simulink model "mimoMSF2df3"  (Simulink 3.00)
settings: Solver=ode45  StartTime=0.0  StopTime=50.0  RelTol=1e-3
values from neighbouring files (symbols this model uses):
  Disturb = Setpoint    [mimo_MSF1DF_sim.m]    (also in mimo_MSF2DF_sim.m)
  K = 1/kpd    [imc2pseucon.m]    (also in imc2pseudo.m)
  Satlb = temp1    [cback.m]    (also in imcmenu.m = str2num(satlbs))
  Satub = temp1    [cback.m]    (also in imcmenu.m = str2num(satubs))
  Setpoint = zeros(1,n)    [mimo_MSF1DF_sim.m]    (also in mimo_MSF2DF_sim.m)
undefined symbols (not defined in the file or in its folder): Ds, input_delay, Kdelay, Ksp, T
libraries: MIMO_lib x14, simulink3 x12

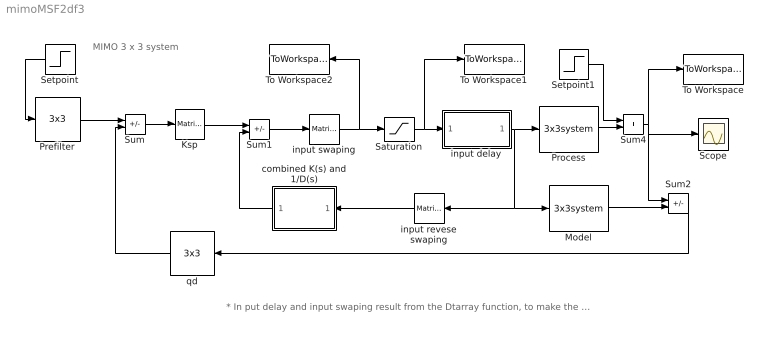
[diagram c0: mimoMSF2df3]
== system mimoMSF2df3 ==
  note: * In put delay and input swaping result from the Dtarray function, to make the system be able to be decoupled.
  note: MIMO 3 x 3 system
  Ksp : simulink3/Math/Matrix Gain  K=Ksp
  Model : MIMO_lib/3x3system  num=Mnum  den=Mden  dead=Mdead
  Prefilter : MIMO_lib/3x3  num=prefilnum  den=prefilden
  Process : MIMO_lib/3x3system  num=Pnum  den=Pden  dead=Pdead
  Saturation : Saturate  UpperLimit=Satub  LowerLimit=Satlb
  Scope : Scope
  Setpoint : Step  Orientation=left  Time=0  Before=0  After=[Setpoint]  SampleTime=0
  Setpoint1 : Step  Time=0  Before=0  After=[Disturb]  SampleTime=0
  Sum : Sum  Inputs=+-  SaturateOnIntegerOverflow=on
  Sum1 : Sum  Inputs=+-  SaturateOnIntegerOverflow=on
  Sum2 : Sum  Inputs=+-  SaturateOnIntegerOverflow=on
  Sum4 : Sum  Inputs=++  SaturateOnIntegerOverflow=on
  To Workspace : ToWorkspace  VariableName=yout  SampleTime=0  SaveFormat=Matrix
  To Workspace1 : ToWorkspace  VariableName=sat_effort  SampleTime=0  SaveFormat=Matrix
  To Workspace2 : ToWorkspace  VariableName=unsat_effort  SampleTime=0  SaveFormat=Matrix
  combined K(s) and 1/D(s) : Subsystem  Orientation=left  mask(ksds){Ksp=Ksp, Ds=Ds, Kdelay=Kdelay, K=K}
      mask prompts: Ds "D(s)"; Kdelay "Bdelay"; K "B*(s)"
  input delay : Subsystem  mask(input delay){input_delay=input_delay}
      mask prompts: input_delay "Input Delay (vector)"
  input revese swaping : simulink3/Math/Matrix Gain  Orientation=left  K=T
  input swaping : simulink3/Math/Matrix Gain  K=inv(T)
  qd : MIMO_lib/3x3  Orientation=left  num=qdnum  den=qdden
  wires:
  Ksp/1 -> Sum1/1
  combined K(s) and 1/D(s)/1(Out1) -> Sum1/2
  Sum/1 -> Ksp/1
  input revese swaping/1 -> combined K(s) and 1/D(s)/1(In1)
  Model/1 -> Sum2/2
  Process/1 -> Sum4/2
  Setpoint1/1 -> Sum4/1
  Sum4/1 -> Sum2/1, To Workspace/1, Scope/1
  input swaping/1 -> Saturation/1, To Workspace2/1
  Sum1/1 -> input swaping/1
  input delay/1(Out1) -> Process/1, Model/1, input revese swaping/1
  Saturation/1 -> input delay/1(In1), To Workspace1/1
  Prefilter/1 -> Sum/1
  Setpoint/1 -> Prefilter/1
  Sum2/1 -> qd/1
  qd/1 -> Sum/2

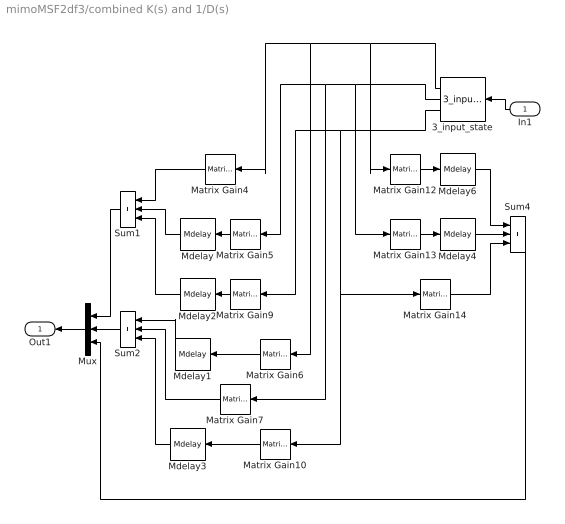
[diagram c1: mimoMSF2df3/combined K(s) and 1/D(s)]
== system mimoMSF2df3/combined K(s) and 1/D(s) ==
  In1 : Inport  Orientation=left  Port=1  PortWidth=-1  SampleTime=-1  DataType=auto
  3_input_state : MIMO_lib/3_input_state  Orientation=left  Ds=Ds
  Matrix Gain10 : simulink3/Math/Matrix Gain  Orientation=left  K="[zeros(1,length(Ds{3})-length(K{2,3}))  K{2,3}]"
  Matrix Gain12 : simulink3/Math/Matrix Gain  K="[zeros(1,length(Ds{1})-length(K{3,1}))  K{3,1}]"
  Matrix Gain13 : simulink3/Math/Matrix Gain  K="[zeros(1,length(Ds{2})-length(K{3,2}))  K{3,2}]"
  Matrix Gain14 : simulink3/Math/Matrix Gain  K="[zeros(1,length(Ds{3})-length(K{3,3}))  K{3,3}]"
  Matrix Gain4 : simulink3/Math/Matrix Gain  Orientation=left  K="[zeros(1,length(Ds{1})-length(K{1,1}))  K{1,1}]"
  Matrix Gain5 : simulink3/Math/Matrix Gain  Orientation=left  K=[zeros(1,length(Ds{2})-length(K{1,2})) K{1,2}]
  Matrix Gain6 : simulink3/Math/Matrix Gain  Orientation=left  K="[zeros(1,length(Ds{1})-length(K{2,1}))  K{2,1}]"
  Matrix Gain7 : simulink3/Math/Matrix Gain  Orientation=left  K="[zeros(1,length(Ds{2})-length(K{2,2}))  K{2,2}]"
  Matrix Gain9 : simulink3/Math/Matrix Gain  Orientation=left  K="[zeros(1,length(Ds{3})-length(K{1,3}))  K{1,3}]"
  Mdelay : MIMO_lib/Mdelay  Orientation=left  Mdelay=Kdelay(1,2)
  Mdelay1 : MIMO_lib/Mdelay  Orientation=left  Mdelay=Kdelay(2,1)
  Mdelay2 : MIMO_lib/Mdelay  Orientation=left  Mdelay=Kdelay(1,3)
  Mdelay3 : MIMO_lib/Mdelay  Orientation=left  Mdelay=Kdelay(2,3)
  Mdelay4 : MIMO_lib/Mdelay  Mdelay=Kdelay(3,2)
  Mdelay6 : MIMO_lib/Mdelay  Mdelay=Kdelay(3,1)
  Mux : Mux  Orientation=left  Inputs=3
  Sum1 : Sum  Orientation=left  Inputs=+++  SaturateOnIntegerOverflow=on
  Sum2 : Sum  Orientation=left  Inputs=+++  SaturateOnIntegerOverflow=on
  Sum4 : Sum  Inputs=+++  SaturateOnIntegerOverflow=on
  Out1 : Outport  Orientation=left  Port=1
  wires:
  Matrix Gain4/1 -> Sum1/1
  Mdelay/1 -> Sum1/2
  Matrix Gain5/1 -> Mdelay/1
  Sum2/1 -> Mux/2
  In1/1 -> 3_input_state/1
  Matrix Gain6/1 -> Mdelay1/1
  Mdelay1/1 -> Sum2/1
  Matrix Gain7/1 -> Sum2/2
  Matrix Gain9/1 -> Mdelay2/1
  Mdelay2/1 -> Sum1/3
  Matrix Gain10/1 -> Mdelay3/1
  3_input_state/3 -> Matrix Gain10/1, Matrix Gain14/1, Matrix Gain9/1
  Mux/1 -> Out1/1
  Mdelay3/1 -> Sum2/3
  Matrix Gain12/1 -> Mdelay6/1
  3_input_state/2 -> Matrix Gain7/1, Matrix Gain5/1, Matrix Gain13/1
  3_input_state/1 -> Matrix Gain6/1, Matrix Gain4/1, Matrix Gain12/1
  Mdelay6/1 -> Sum4/1
  Matrix Gain13/1 -> Mdelay4/1
  Mdelay4/1 -> Sum4/2
  Matrix Gain14/1 -> Sum4/3
  Sum4/1 -> Mux/3
  Sum1/1 -> Mux/1

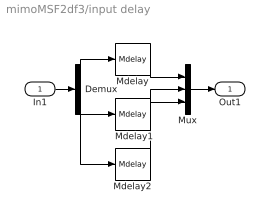
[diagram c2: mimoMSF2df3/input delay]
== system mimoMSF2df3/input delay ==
  In1 : Inport  Port=1  PortWidth=-1  SampleTime=-1  DataType=auto
  Demux : Demux  Outputs=3
  Mdelay : MIMO_lib/Mdelay  Mdelay=input_delay(1)
  Mdelay1 : MIMO_lib/Mdelay  Mdelay=input_delay(2)
  Mdelay2 : MIMO_lib/Mdelay  Mdelay=input_delay(3)
  Mux : Mux  Inputs=3
  Out1 : Outport  Port=1
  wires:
  Mux/1 -> Out1/1
  In1/1 -> Demux/1
  Demux/1 -> Mdelay/1
  Demux/2 -> Mdelay1/1
  Mdelay/1 -> Mux/1
  Mdelay1/1 -> Mux/2
  Demux/3 -> Mdelay2/1
  Mdelay2/1 -> Mux/3
